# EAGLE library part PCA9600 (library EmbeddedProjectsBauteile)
Dual bidirectional I²C Bus Buffer
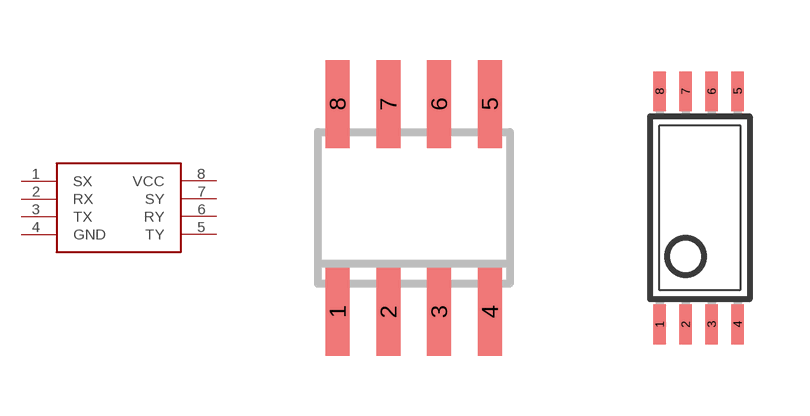
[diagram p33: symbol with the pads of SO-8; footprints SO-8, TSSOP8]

Designator prefix IC

## PCA9600D  [SO-8]
1  SX
2  RX
3  TX
4  GND
5  TY
6  RY
7  SY
8  VCC  pwr

## PCA9600DP  [TSSOP8]
Pads as for SO-8

## Footprint SO-8 (pad centres in mm)
smd 0.6 x 2.2: 1 -1.905,-2.6; 2 -0.635,-2.6; 3 0.635,-2.6; 4 1.905,-2.6; 5 1.905,2.6; 6 0.635,2.6; 7 -0.635,2.6; 8 -1.905,2.6

## Footprint TSSOP8 (pad centres in mm)
smd 0.305 x 0.991: 1 -1.005,-2.918; 2 -0.355,-2.918; 3 0.295,-2.918; 4 0.945,-2.918; 5 0.945,2.918; 6 0.295,2.918; 7 -0.355,2.918; 8 -1.005,2.918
